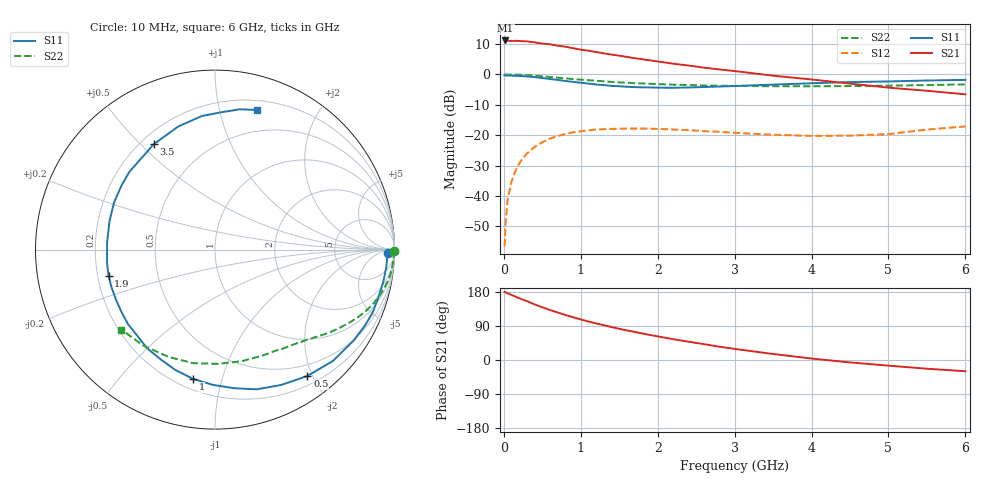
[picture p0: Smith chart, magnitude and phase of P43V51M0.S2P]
! SIEMENS Small Signal Semiconductors
! BFP182
! Si NPN RF Bipolar Junction Transistor in SOT143
! VCE = 3.5 V  IC = 1 mA
! Common Emitter S-Parameters:  March  1996
# GHz  S  MA  R  50
!  f  S11  S21  S12  S22
! GHz  MAG  ANG  MAG  ANG  MAG  ANG  MAG  ANG
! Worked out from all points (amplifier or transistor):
!   36 points, 10 MHz to 6 GHz, reference 50 ohm
!   highest |S21| = 11.2 dB at 20 MHz (marker M1)
!   |S21| within 3 dB of that: start of sweep to 996.2 MHz
!   unconditionally stable (mu >= 1): 2.605 GHz to end of sweep
!   at 250 MHz: K = 0.10, MSG = 19.2 dB, |S12| = -27.5 dB
!   at 1.4 GHz: K = 0.53, MSG = 12.2 dB, |S12| = -17.9 dB
!   at 6 GHz: K = 1.06, MAG = 3.8 dB, |S12| = -17.1 dB
!   S11 on the Smith chart (normalised r, x): 10 MHz: 45, -22; 500 MHz: 0.33, -1.93; 1 GHz: 0.26, -0.81; 1.9 GHz: 0.24, -0.11; 3.5 GHz: 0.25, +0.55; 6 GHz: 0.29, +1.31
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0.01  0.965 -1.0  3.566 179.5  0.0015 87.7  0.9976 -0.4
0.02  0.9608 -2.3  3.615 179.0  0.0032 96.9  0.9958 -0.8
0.05  0.9596 -5.7  3.595 175.8  0.009 88.9  0.9969 -2.0
0.1  0.9547 -10.9  3.548 171.6  0.0174 82.8  0.9936 -4.1
0.15  0.9482 -16.9  3.566 167.4  0.0259 79.3  0.9913 -6.2
0.3  0.9244 -33.0  3.493 155.4  0.05 69.6  0.9715 -12.0
0.4  0.9038 -43.3  3.364 146.8  0.0642 63.3  0.9521 -15.7
0.5  0.8724 -53.8  3.216 139.1  0.077 57.1  0.9307 -19.1
0.6  0.8398 -63.8  3.129 132.0  0.0883 51.5  0.907 -22.2
0.8  0.7794 -82.2  2.852 118.8  0.1047 41.6  0.8606 -27.6
1  0.7306 -99.7  2.554 107.1  0.1162 32.9  0.8198 -32.1
1.1  0.7058 -108.3  2.452 101.5  0.1207 29.3  0.8015 -34.2
1.3  0.6675 -124.5  2.222 91.8  0.126 22.2  0.7687 -37.9
1.5  0.6384 -139.3  2.034 82.3  0.1278 16.9  0.7398 -41.3
1.9  0.6109 -166.2  1.7 66.1  0.1281 8.1  0.7005 -47.6
2.2  0.6027 176.0  1.499 54.9  0.124 3.6  0.6782 -52.3
2.8  0.6314 145.6  1.209 35.2  0.114 -2.0  0.6518 -62.5
3.5  0.6791 120.2  0.953 15.8  0.1018 -1.9  0.6391 -76.7
4  0.7156 106.7  0.825 3.9  0.0975 2.7  0.6368 -88.2
4.5  0.748 95.6  0.707 -6.4  0.0985 7.3  0.644 -100.7
5.5  0.7939 80.0  0.538 -23.0  0.1238 16.5  0.6676 -126.7
6  0.8124 73.2  0.471 -29.7  0.1397 15.3  0.6859 -139.5
